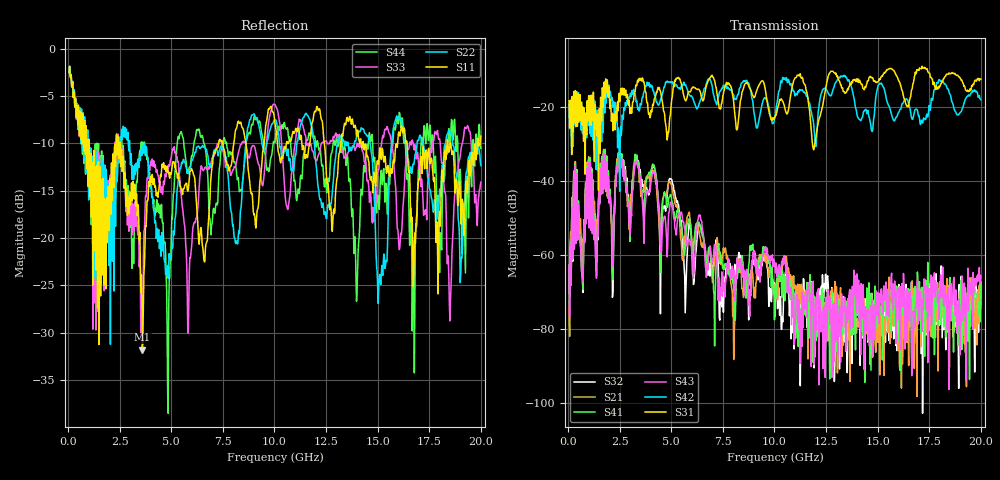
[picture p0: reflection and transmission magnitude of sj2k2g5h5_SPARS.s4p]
! FILE: E:\users\goganessyan\GBX_Backplane\FR408_backplane\1m_OUTBOUND_FEXT\sj2k2g5h5_SPARS.s4p
# MHZ S RI R 50.00
! FREQ  S11  S12  S13  S14
!  S21  S22  S23  S24
!  S31  S32  S33  S34
!  S41  S42  S43  S44
!  REAL  IMAG  REAL  IMAG  REAL  IMAG  REAL  IMAG
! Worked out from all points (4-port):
!   799 points, 50 MHz to 20 GHz, reference 50 ohm
!   strongest paths, dB at 50 MHz, 5.025 GHz, 10.03 GHz, 15.03 GHz, 20 GHz:
!     S31: -18.3, -17.8, -22.5, -13.2, -12.5
!     S42: -19.4, -13.5, -22.6, -14.1, -18.1
!     S43: -63.1, -46.9, -62.3, -70.8, -65.6
!     S41: -73.3, -45.5, -70.5, -76.8, -67.2
!     S21: -74.0, -41.4, -76.7, -73.5, -73.3
!     S32: -62.8, -39.7, -68.2, -78.6, -71.8
!   lowest |S11| = -31.8 dB at 3.6 GHz (marker M1), VSWR 1.05, Z = 50.8 + j2.45 ohm
!   |S11| at or under -10 dB: 2.505 GHz to 7.302 GHz (4.798 GHz wide, 97.8 % of centre); 14.31 GHz to 15.96 GHz (1.656 GHz wide, 10.9 % of centre); 16.43 GHz to 18.36 GHz (1.938 GHz wide, 11.1 % of centre)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
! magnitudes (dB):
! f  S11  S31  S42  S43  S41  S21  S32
! 50 MHz  -2.5  -18.3  -19.4  -63.1  -73.3  -74.0  -62.8
! 350 MHz  -5.2  -15.6  -15.7  -35.9  -35.4  -34.8  -34.9
! 675 MHz  -10.1  -24.9  -23.9  -63.8  -66.0  -55.7  -61.6
! 3.6 GHz  -31.8  -12.2  -17.4  -45.5  -44.5  -44.1  -41.3
! 4.85 GHz  -13.1  -26.7  -13.3  -51.3  -46.2  -41.1  -41.1
! 7.4 GHz  -9.7  -20.4  -15.6  -70.1  -61.9  -62.5  -71.8
! 20 GHz  -9.2  -12.5  -18.1  -65.6  -67.2  -73.3  -71.8
